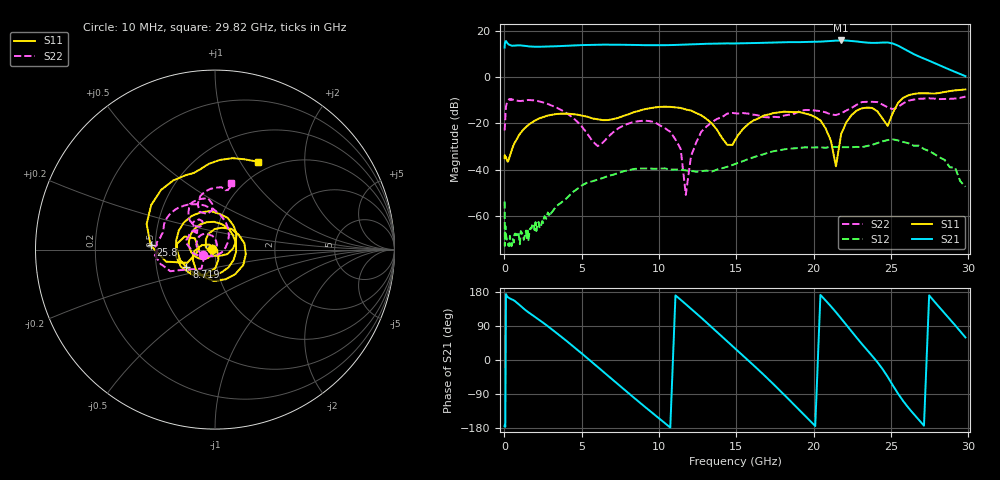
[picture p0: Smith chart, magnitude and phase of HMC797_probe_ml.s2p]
! Hittite Microwave Corporation
! 20 Alpha Road
! Chelmsford, MA 01824
! http://www.hittite.com
! Tel: 978-250-3343
! Fax: 978-250-3373
! Device:  HMC797
! Description: GaAs HEMT MMIC Medium Power Amplifier
! Frequency:  DC - 22.00 GHz
! Package:  DIE
! Ports:  2 RF, 2 DC
!  Pad 1 = RF in  = Port 1
!  Pad 2 = Vgg2
!  Pad 3 = ACG1
!  Pad 4 = ACG2
!  Pad 5 = DC and RF Out = Port 2
!  Pad 6 = ACG3
!  Pad 7 = ACG4
!  Pad 8 = Vgg1
! Voltages:  Vdd  = 10.00 Volts, Idd  = 399.9 mA
!  Vgg1 = -1.26 Volts, Igg1 =  -6.3 mA
!  Vgg2 =  3.50 Volts, Igg2 =  -7.2 uA
! Data:  The device was measured using G-S-G Probes on a microstrip
!  alumina launch with 1 mil wirebonds of approximately 20 mils
!  in length to the RF ports. The microstrip launch is 280 mils long.
!  Data was collected using an calibrated network analyzer.
!  The reference plane is the pads on the microstrip launch.
! Misc:  Validation Unit 6
! Date Measured:  2010-03-04
! Date:  2010-07-20  MJV
! Note:
!  Hittite supplies this data as a sample of measured data at the package pin for
!  for this package product.  Your particular data for this product may vary.
!  Data was taken at 25 degrees C.
!  Hittite reserves the right to change this data at anytime.
!  Data was taken at 25 degrees C.
# GHZ S DB R 50.0
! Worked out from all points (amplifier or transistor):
!   140 points, 10 MHz to 29.82 GHz, reference 50 ohm
!   highest |S21| = 15.9 dB at 21.78 GHz (marker M1)
!   |S21| within 3 dB of that: 10.85 MHz to 25.67 GHz (25.66 GHz wide, 200 % of centre)
!   unconditionally stable (mu >= 1): start of sweep to end of sweep
!   at 1.206 GHz: K = 247.82, MAG = 14.1 dB, |S12| = -68.5 dB
!   at 6.709 GHz: K = 13.34, MAG = 14.1 dB, |S12| = -42.7 dB
!   at 29.82 GHz: K = 66.42, MAG = 2.7 dB, |S12| = -47.3 dB
!   S11 on the Smith chart (normalised r, x): 10 MHz: 0.97, +0.00; 8.719 GHz: 0.71, -0.15; 25.8 GHz: 0.47, +0.03; 29.82 GHz: 0.86, +1.19
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0.01  -35.01 174.3  12.79 -174.6  -53.74 133.6  -23.05 -156.5
0.0997  -34.51 177.7  15.64 173.9  -68.13 21.4  -12.73 -150.1
2.5515  -17.11 179.2  13.22 96.8  -61.06 83.5  -11.02 115.8
5.03425  -16.64 75.4  13.89 16.1  -46.72 -19.5  -21.56 30.4
7.043951  -18.10 -52.9  14.06 -53.6  -42.19 -68.9  -23.78 -149.8
8.718701  -14.53 -148.3  13.91 -111.3  -39.49 -110.5  -19.01 152.8
10.0585  -12.84 152.2  13.80 -155.9  -39.52 -142.9  -20.85 112.2
11.3983  -13.29 96.4  14.04 159.1  -40.00 177.9  -30.95 65.7
13.07305  -18.09 20.6  14.44 99.0  -40.37 110.1  -21.35 -153.0
15.08275  -25.36 163.3  14.62 24.5  -37.12 20.5  -15.72 154.5
16.42255  -17.88 72.2  14.81 -25.5  -33.94 -25.0  -16.51 133.7
17.76235  -15.21 -8.6  15.09 -78.2  -31.65 -67.6  -17.30 137.5
18.7672  -15.11 -69.7  15.16 -119.2  -30.79 -98.9  -15.77 134.3
20.107  -17.28 -154.2  15.28 -174.3  -30.38 -145.1  -14.43 118.0
21.78175  -24.64 -70.5  15.89 109.5  -30.29 140.3  -15.58 128.9
22.45165  -16.42 -112.2  15.67 75.6  -30.28 101.8  -13.30 130.9
23.79145  -13.30 171.8  14.83 10.8  -29.27 29.0  -10.65 106.4
24.46135  -17.87 150.9  14.98 -23.8  -27.73 -4.7  -11.84 93.5
25.13125  -15.35 -154.5  14.56 -67.2  -26.89 -39.9  -13.83 102.2
25.80115  -8.87 176.0  12.42 -108.6  -28.02 -75.3  -11.31 110.8
27.81085  -7.07 105.4  6.13 154.4  -33.21 -143.4  -9.28 81.5
29.82055  -5.29 64.1  0.46 59.6  -47.35 128.7  -8.40 76.3
